| TEXAS INSTRUMENTS INCORPORATED
| Standard Linear and Logic Group
| IBIS Model of SN74CBT16211C
| 24-BIT FET BUS SWITCH WITH -2-V UNDERSHOOT PROTECTION
| This file contains package information for the following:
|  TSSOP 56-pin (DGG) package as [Component] CBT16211C_DGG
|  TVSOP 56-pin (DGV) package as [Component] CBT16211C_DGV
|  SSOP 56-pin (DL) package as [Component] CBT16211C_DL
| This device can be powered at the following Vccs:
|  5 volt Vcc
|  4 volt Vcc
| This file provides unique models under the [Model Selector] for each Vcc.
| For operation at a specific Vcc, select the appropriate model after each
| [Model Selector] keyword.
[IBIS Ver]   3.2
[Comment char]  |_char
[File Name]   sn74cbt16211c.ibs
[File Rev]   1.1 | a_die
[Date]   June 24, 2003
[Source]   Data created from TI-SPICE simulations at TI-SLL.
[Notes]   The following is an IBIS list for the SN74CBT16211C.
   Please contact sllibis@ti.com with questions and
   comments concerning SLL IBIS models.
   - Non-monotonic data due to FET characteristics.
   - C_comp values are taken at a different test condition than
   the Cio in data sheet.
   - Power-clamp data has been deleted since there is no
   power-clamp diode in the device.
[Disclaimer] Property of Texas Instruments Incorporated. Unauthorized
   reproduction and/or distribution is strictly prohibited.
   This product is protected under copyright law.
   Created 2003,(C) Copyright 2003, Texas Instruments
   Incorporated, All Rights Reserved
   UNLESS THERE IS A SIGNED, WRITTEN AGREEMENT TO THE
   CONTRARY, TEXAS INSTRUMENTS (TI) IS PROVIDING THE IBIS
   MODELS AND WITHOUT ANY WARRANTY, EXPRESSED OR
   IMPLIED. TI assumes no liability for:
   1) the accuracy of the IBIS models provided to your
   company;
   2) the proper functioning of these IBIS Models in your
   design or for any resulting applications; or
   3) infringement of patents, copyrights or intellectual
   property rights resulting from your use of these IBIS
   models.
   TI provides IBIS Models as a service to our customers.
   You and your company shall not distribute, sell or give
   these models to anyone else without prior written
   permission from TI.
   TI reserves the right to make changes to our products or
   to discontinue any semiconductor product or service
   without notice, and advises our customers to obtain the
   latest version of relevant information to verify, before
   placing orders, that the information being relied on is
   current.
   Please be aware that your receipt and use of the IBIS
   information provided shall serve as acceptance of these
   terms and conditions. If you do not accept these terms,
   you should return or destroy the IBIS models and any
   other accompanying information immediately.
| Component CBT16211C_DGG 56-pin TSSOP
[Component]   CBT16211C_DGG
[Manufacturer]   Texas Instruments, Inc.
[Package]
|   typ   min   max
R_pkg   5.400e-02   4.000e-02   8.300e-02
L_pkg   3.546e-09   2.838e-09   5.045e-09
C_pkg   5.580e-13   4.120e-13   7.380e-13
[Pin]   signal_name   model_name   R_pin   L_pin   C_pin
1   NC   NC   7.600e-02   5.003e-09   7.120e-13
2   1A1   CBT16211C_IO   7.600e-02   4.539e-09   7.230e-13
3   1A2   CBT16211C_IO   8.300e-02   4.357e-09   7.080e-13
4   1A3   CBT16211C_IO   4.200e-02   3.999e-09   6.830e-13
5   1A4   CBT16211C_IO   4.200e-02   3.806e-09   6.700e-13
6   1A5   CBT16211C_IO   4.300e-02   3.603e-09   6.160e-13
7   1A6   CBT16211C_IO   4.400e-02   3.440e-09   5.520e-13
8   GND   GND   4.600e-02   3.306e-09   5.090e-13
9   1A7   CBT16211C_IO   4.700e-02   3.194e-09   4.820e-13
10   1A8   CBT16211C_IO   4.800e-02   3.088e-09   4.630e-13
11   1A9   CBT16211C_IO   5.000e-02   2.987e-09   4.350e-13
12   1A10   CBT16211C_IO   5.100e-02   2.910e-09   4.230e-13
13   1A11   CBT16211C_IO   5.200e-02   2.894e-09   4.220e-13
14   1A12   CBT16211C_IO   5.300e-02   2.840e-09   4.220e-13
15   2A1   CBT16211C_IO   5.300e-02   2.850e-09   4.230e-13
16   2A2   CBT16211C_IO   5.200e-02   2.886e-09   4.210e-13
17   VCC   POWER   5.100e-02   2.883e-09   4.190e-13
18   2A3   CBT16211C_IO   5.000e-02   2.941e-09   4.300e-13
19   GND   GND   4.900e-02   3.031e-09   4.570e-13
20   2A4   CBT16211C_IO   4.700e-02   3.131e-09   4.760e-13
21   2A5   CBT16211C_IO   4.600e-02   3.244e-09   5.030e-13
22   2A6   CBT16211C_IO   4.400e-02   3.387e-09   5.500e-13
23   2A7   CBT16211C_IO   4.300e-02   3.566e-09   6.320e-13
24   2A8   CBT16211C_IO   4.200e-02   3.801e-09   6.870e-13
25   2A9   CBT16211C_IO   4.100e-02   3.961e-09   6.870e-13
26   2A10   CBT16211C_IO   8.100e-02   4.291e-09   7.110e-13
27   2A11   CBT16211C_IO   7.600e-02   4.561e-09   7.380e-13
28   2A12   CBT16211C_IO   7.500e-02   5.045e-09   7.240e-13
29   2B12   CBT16211C_IO   7.300e-02   5.020e-09   7.140e-13
30   2B11   CBT16211C_IO   7.400e-02   4.532e-09   7.200e-13
31   2B10   CBT16211C_IO   8.300e-02   4.336e-09   7.080e-13
32   2B9   CBT16211C_IO   4.000e-02   3.957e-09   6.840e-13
33   2B8   CBT16211C_IO   4.200e-02   3.789e-09   6.800e-13
34   2B7   CBT16211C_IO   4.300e-02   3.540e-09   6.240e-13
35   2B6   CBT16211C_IO   4.400e-02   3.361e-09   5.460e-13
36   2B5   CBT16211C_IO   4.600e-02   3.222e-09   4.980e-13
37   2B4   CBT16211C_IO   4.700e-02   3.110e-09   4.710e-13
38   GND   GND   4.800e-02   3.012e-09   4.510e-13
39   2B3   CBT16211C_IO   5.000e-02   2.934e-09   4.230e-13
40   2B2   CBT16211C_IO   5.100e-02   2.879e-09   4.120e-13
41   2B1   CBT16211C_IO   5.200e-02   2.883e-09   4.130e-13
42   1B12   CBT16211C_IO   5.300e-02   2.847e-09   4.170e-13
43   1B11   CBT16211C_IO   5.300e-02   2.838e-09   4.170e-13
44   1B10   CBT16211C_IO   5.200e-02   2.887e-09   4.160e-13
45   1B9   CBT16211C_IO   5.100e-02   2.897e-09   4.160e-13
46   1B8   CBT16211C_IO   5.000e-02   2.965e-09   4.270e-13
47   1B7   CBT16211C_IO   4.800e-02   3.047e-09   4.550e-13
48   1B6   CBT16211C_IO   4.700e-02   3.138e-09   4.740e-13
49   GND   GND   4.600e-02   3.250e-09   5.030e-13
50   1B5   CBT16211C_IO   4.400e-02   3.390e-09   5.500e-13
51   1B4   CBT16211C_IO   4.300e-02   3.546e-09   6.260e-13
52   1B3   CBT16211C_IO   4.200e-02   3.783e-09   6.860e-13
53   1B2   CBT16211C_IO   4.000e-02   3.955e-09   6.820e-13
54   1B1   CBT16211C_IO   8.300e-02   4.330e-09   7.010e-13
55   2NOE   CBT16211C_IN   7.700e-02   4.562e-09   7.240e-13
56   1NOE   CBT16211C_IN   7.500e-02   5.029e-09   7.120e-13
| Component CBT16211C_DGV 56-pin TVSOP
[Component]   CBT16211C_DGV
[Manufacturer]   Texas Instruments, Inc.
[Package]
|   typ   min   max
R_pkg   6.300e-02   5.000e-02   8.400e-02
L_pkg   2.945e-09   2.394e-09   3.939e-09
C_pkg   3.910e-13   2.710e-13   5.880e-13
[Pin]   signal_name   model_name   R_pin   L_pin   C_pin
1   NC   NC   6.800e-02   3.933e-09   5.880e-13
2   1A1   CBT16211C_IO   6.800e-02   3.568e-09   5.870e-13
3   1A2   CBT16211C_IO   7.600e-02   3.464e-09   5.150e-13
4   1A3   CBT16211C_IO   8.400e-02   3.444e-09   4.590e-13
5   1A4   CBT16211C_IO   8.100e-02   3.277e-09   4.270e-13
6   1A5   CBT16211C_IO   7.400e-02   3.136e-09   3.870e-13
7   1A6   CBT16211C_IO   6.900e-02   2.970e-09   4.010e-13
8   GND   GND   5.000e-02   2.785e-09   3.790e-13
9   1A7   CBT16211C_IO   5.100e-02   2.685e-09   3.200e-13
10   1A8   CBT16211C_IO   5.300e-02   2.611e-09   3.160e-13
11   1A9   CBT16211C_IO   5.300e-02   2.495e-09   2.970e-13
12   1A10   CBT16211C_IO   5.300e-02   2.435e-09   2.920e-13
13   1A11   CBT16211C_IO   5.500e-02   2.412e-09   2.850e-13
14   1A12   CBT16211C_IO   5.600e-02   2.401e-09   2.730e-13
15   2A1   CBT16211C_IO   5.500e-02   2.401e-09   2.730e-13
16   2A2   CBT16211C_IO   5.500e-02   2.399e-09   2.840e-13
17   VCC   POWER   5.400e-02   2.406e-09   2.890e-13
18   2A3   CBT16211C_IO   5.300e-02   2.450e-09   2.930e-13
19   GND   GND   5.100e-02   2.544e-09   3.110e-13
20   2A4   CBT16211C_IO   5.100e-02   2.626e-09   3.150e-13
21   2A5   CBT16211C_IO   5.000e-02   2.727e-09   3.690e-13
22   2A6   CBT16211C_IO   6.500e-02   2.903e-09   3.930e-13
23   2A7   CBT16211C_IO   7.500e-02   3.091e-09   3.860e-13
24   2A8   CBT16211C_IO   8.200e-02   3.272e-09   4.280e-13
25   2A9   CBT16211C_IO   8.200e-02   3.393e-09   4.570e-13
26   2A10   CBT16211C_IO   7.300e-02   3.380e-09   5.080e-13
27   2A11   CBT16211C_IO   7.100e-02   3.577e-09   5.800e-13
28   2A12   CBT16211C_IO   6.800e-02   3.937e-09   5.740e-13
29   2B12   CBT16211C_IO   6.900e-02   3.923e-09   5.690e-13
30   2B11   CBT16211C_IO   6.400e-02   3.536e-09   5.740e-13
31   2B10   CBT16211C_IO   7.600e-02   3.428e-09   5.170e-13
32   2B9   CBT16211C_IO   8.100e-02   3.395e-09   4.680e-13
33   2B8   CBT16211C_IO   8.000e-02   3.255e-09   4.310e-13
34   2B7   CBT16211C_IO   7.100e-02   3.064e-09   3.860e-13
35   2B6   CBT16211C_IO   6.100e-02   2.878e-09   3.890e-13
36   2B5   CBT16211C_IO   5.000e-02   2.710e-09   3.630e-13
37   2B4   CBT16211C_IO   5.000e-02   2.606e-09   3.110e-13
38   GND   GND   5.200e-02   2.534e-09   3.060e-13
39   2B3   CBT16211C_IO   5.200e-02   2.439e-09   2.890e-13
40   2B2   CBT16211C_IO   5.300e-02   2.399e-09   2.860e-13
41   2B1   CBT16211C_IO   5.500e-02   2.394e-09   2.820e-13
42   1B12   CBT16211C_IO   5.500e-02   2.398e-09   2.710e-13
43   1B11   CBT16211C_IO   5.600e-02   2.396e-09   2.710e-13
44   1B10   CBT16211C_IO   5.400e-02   2.402e-09   2.830e-13
45   1B9   CBT16211C_IO   5.400e-02   2.423e-09   2.880e-13
46   1B8   CBT16211C_IO   5.300e-02   2.474e-09   2.920e-13
47   1B7   CBT16211C_IO   5.100e-02   2.569e-09   3.090e-13
48   1B6   CBT16211C_IO   5.100e-02   2.638e-09   3.130e-13
49   GND   GND   5.100e-02   2.742e-09   3.660e-13
50   1B5   CBT16211C_IO   6.400e-02   2.917e-09   3.900e-13
51   1B4   CBT16211C_IO   7.400e-02   3.083e-09   3.830e-13
52   1B3   CBT16211C_IO   8.100e-02   3.249e-09   4.300e-13
53   1B2   CBT16211C_IO   8.300e-02   3.400e-09   4.550e-13
54   1B1   CBT16211C_IO   7.500e-02   3.427e-09   5.050e-13
55   2NOE   CBT16211C_IN   7.100e-02   3.585e-09   5.780e-13
56   1NOE   CBT16211C_IN   6.900e-02   3.939e-09   5.810e-13
| Component CBT16211C_DL 56-pin SSOP
[Component]   CBT16211C_DL
[Manufacturer]   Texas Instruments, Inc.
[Package]
|   typ   min   max
R_pkg   5.500e-02   4.800e-02   6.700e-02
L_pkg   6.539e-09   4.803e-09   9.746e-09
C_pkg   8.570e-13   5.000e-13   1.351e-12
[Pin]   signal_name   model_name   R_pin   L_pin   C_pin
1   NC   NC   6.400e-02   9.646e-09   1.202e-12
2   1A1   CBT16211C_IO   5.900e-02   8.723e-09   1.348e-12
3   1A2   CBT16211C_IO   5.900e-02   8.139e-09   1.223e-12
4   1A3   CBT16211C_IO   5.600e-02   7.554e-09   1.088e-12
5   1A4   CBT16211C_IO   5.400e-02   6.991e-09   9.660e-13
6   1A5   CBT16211C_IO   5.300e-02   6.659e-09   9.730e-13
7   1A6   CBT16211C_IO   5.500e-02   6.321e-09   9.050e-13
8   GND   GND   5.600e-02   5.942e-09   7.130e-13
9   1A7   CBT16211C_IO   5.700e-02   5.768e-09   6.780e-13
10   1A8   CBT16211C_IO   5.400e-02   5.459e-09   6.310e-13
11   1A9   CBT16211C_IO   5.100e-02   5.224e-09   6.380e-13
12   1A10   CBT16211C_IO   4.800e-02   5.088e-09   6.010e-13
13   1A11   CBT16211C_IO   5.000e-02   5.021e-09   5.180e-13
14   1A12   CBT16211C_IO   5.100e-02   4.803e-09   5.000e-13
15   2A1   CBT16211C_IO   5.100e-02   4.803e-09   5.000e-13
16   2A2   CBT16211C_IO   5.000e-02   5.021e-09   5.180e-13
17   VCC   POWER   4.800e-02   5.088e-09   6.010e-13
18   2A3   CBT16211C_IO   5.100e-02   5.224e-09   6.380e-13
19   GND   GND   5.400e-02   5.459e-09   6.310e-13
20   2A4   CBT16211C_IO   5.700e-02   5.768e-09   6.770e-13
21   2A5   CBT16211C_IO   5.500e-02   5.942e-09   7.150e-13
22   2A6   CBT16211C_IO   5.500e-02   6.321e-09   9.070e-13
23   2A7   CBT16211C_IO   5.300e-02   6.659e-09   9.720e-13
24   2A8   CBT16211C_IO   5.400e-02   6.991e-09   9.660e-13
25   2A9   CBT16211C_IO   5.600e-02   7.554e-09   1.087e-12
26   2A10   CBT16211C_IO   5.900e-02   8.139e-09   1.223e-12
27   2A11   CBT16211C_IO   5.900e-02   8.727e-09   1.351e-12
28   2A12   CBT16211C_IO   6.700e-02   9.746e-09   1.210e-12
29   2B12   CBT16211C_IO   6.300e-02   9.630e-09   1.203e-12
30   2B11   CBT16211C_IO   6.000e-02   8.751e-09   1.349e-12
31   2B10   CBT16211C_IO   6.000e-02   8.184e-09   1.224e-12
32   2B9   CBT16211C_IO   5.600e-02   7.543e-09   1.087e-12
33   2B8   CBT16211C_IO   5.400e-02   7.005e-09   9.690e-13
34   2B7   CBT16211C_IO   5.600e-02   6.714e-09   9.750e-13
35   2B6   CBT16211C_IO   5.800e-02   6.384e-09   9.090e-13
36   2B5   CBT16211C_IO   5.700e-02   5.976e-09   7.170e-13
37   2B4   CBT16211C_IO   5.700e-02   5.743e-09   6.770e-13
38   GND   GND   5.400e-02   5.468e-09   6.310e-13
39   2B3   CBT16211C_IO   5.500e-02   5.329e-09   6.440e-13
40   2B2   CBT16211C_IO   5.200e-02   5.189e-09   6.060e-13
41   2B1   CBT16211C_IO   5.200e-02   5.053e-09   5.190e-13
42   1B12   CBT16211C_IO   5.200e-02   4.825e-09   5.020e-13
43   1B11   CBT16211C_IO   5.400e-02   4.897e-09   5.060e-13
44   1B10   CBT16211C_IO   5.200e-02   5.093e-09   5.210e-13
45   1B9   CBT16211C_IO   5.100e-02   5.179e-09   6.080e-13
46   1B8   CBT16211C_IO   5.400e-02   5.314e-09   6.450e-13
47   1B7   CBT16211C_IO   5.500e-02   5.511e-09   6.320e-13
48   1B6   CBT16211C_IO   5.700e-02   5.770e-09   6.770e-13
49   GND   GND   5.600e-02   5.956e-09   7.160e-13
50   1B5   CBT16211C_IO   5.500e-02   6.320e-09   9.050e-13
51   1B4   CBT16211C_IO   5.200e-02   6.621e-09   9.680e-13
52   1B3   CBT16211C_IO   5.300e-02   6.974e-09   9.660e-13
53   1B2   CBT16211C_IO   5.700e-02   7.571e-09   1.089e-12
54   1B1   CBT16211C_IO   5.700e-02   8.097e-09   1.219e-12
55   2NOE   CBT16211C_IN   5.900e-02   8.723e-09   1.349e-12
56   1NOE   CBT16211C_IN   6.100e-02   9.560e-09   1.199e-12
[Series Switch Groups]
| Function Group States
On  1 /   | 1A1-1A12->1B1-1B12 1NOE Low
On  2 /   | 2A1-2A12->2B1-2B12 2NOE Low
On  1 2 /   | ENABLE BOTH   |
[Series Pin Mapping]   pin_2   model_name   function_table_group
2   54   CBT16211C_IO_50_S   1
| 2   54   CBT16211C_IO_40_S   1
3   53   CBT16211C_IO_50_S   1
| 3   53   CBT16211C_IO_40_S   1
4   52   CBT16211C_IO_50_S   1
| 4   52   CBT16211C_IO_40_S   1
5   51   CBT16211C_IO_50_S   1
| 5   51   CBT16211C_IO_40_S   1
6   50   CBT16211C_IO_50_S   1
| 6   50   CBT16211C_IO_40_S   1
7   48   CBT16211C_IO_50_S   1
| 7   48   CBT16211C_IO_40_S   1
9   47   CBT16211C_IO_50_S   1
| 9   47   CBT16211C_IO_40_S   1
10   46   CBT16211C_IO_50_S   1
| 10   46   CBT16211C_IO_40_S   1
11   45   CBT16211C_IO_50_S   1
| 11   45   CBT16211C_IO_40_S   1
12   44   CBT16211C_IO_50_S   1
| 12   44   CBT16211C_IO_40_S   1
13   43   CBT16211C_IO_50_S   1
| 13   43   CBT16211C_IO_40_S   1
14   42   CBT16211C_IO_50_S   1
| 14   42   CBT16211C_IO_40_S   1
15   41   CBT16211C_IO_50_S   2
| 15   41   CBT16211C_IO_40_S   2
16   40   CBT16211C_IO_50_S   2
| 16   40   CBT16211C_IO_40_S   2
18   39   CBT16211C_IO_50_S   2
| 18   39   CBT16211C_IO_40_S   2
21   36   CBT16211C_IO_50_S   2
| 21   36   CBT16211C_IO_40_S   2
22   35   CBT16211C_IO_50_S   2
| 22   35   CBT16211C_IO_40_S   2
23   34   CBT16211C_IO_50_S   2
| 23   34   CBT16211C_IO_40_S   2
24   33   CBT16211C_IO_50_S   2
| 24   33   CBT16211C_IO_40_S   2
25   32   CBT16211C_IO_50_S   2
| 25   32   CBT16211C_IO_40_S   2
26   31   CBT16211C_IO_50_S   2
| 26   31   CBT16211C_IO_40_S   2
27   30   CBT16211C_IO_50_S   2
| 27   30   CBT16211C_IO_40_S   2
28   29   CBT16211C_IO_50_S   2
| 28   29   CBT16211C_IO_40_S   2
| Model CBT16211C_IN
[Model Selector]   CBT16211C_IN
CBT16211C_IN_50   5 volt Vcc
CBT16211C_IN_40   4 volt Vcc
| Model CBT16211C_IO
[Model Selector]   CBT16211C_IO
CBT16211C_IO_50   5 volt Vcc
CBT16211C_IO_40   4 volt Vcc
| Model CBT16211C_IO_S
[Model Selector]   CBT16211C_IO_S
CBT16211C_IO_50_S   5 volt Vcc
CBT16211C_IO_40_S   4 volt Vcc
[Model]   CBT16211C_IO_50_S
Model_type  Series_switch
| variable   typ   min   max
C_comp   0   0   0
[Temperature Range]   40   100   -40
| Ambient temperature   25   85   -40
[Voltage range]   5   4.5   5.5
[On]
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[Off]
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[Model]   CBT16211C_IO_40_S
Model_type  Series_switch
| variable   typ   min   max
C_comp   0   0   0
[Temperature Range]   40   100   -40
| Ambient temperature   25   85   -40
[Voltage range]   4   4   4
[On]
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[Off]
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| Models and submodels in the file (6): CBT16211C_IN_50 (Input), CBT16211C_IN_40 (Input), CBT16211C_IO_50_S (Series_switch), CBT16211C_IO_50 (Terminator), CBT16211C_IO_40_S (Series_switch), CBT16211C_IO_40 (Terminator)
